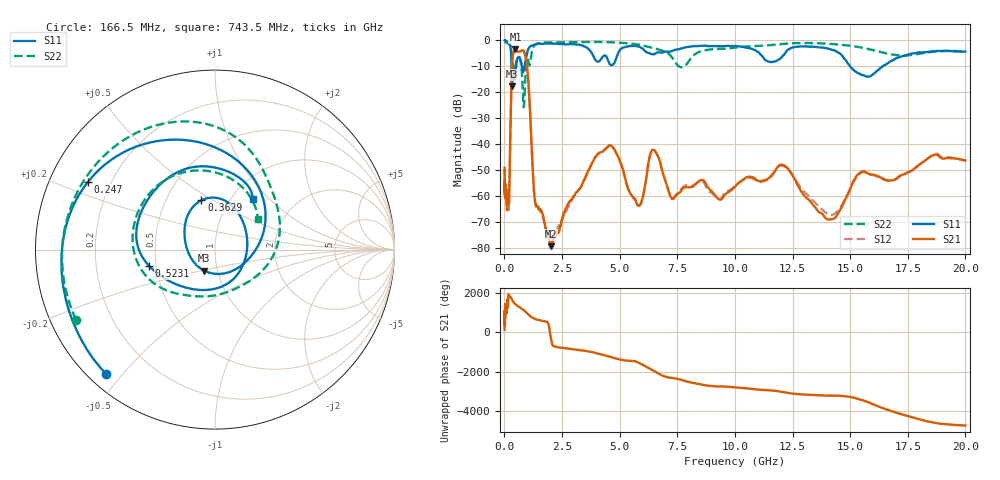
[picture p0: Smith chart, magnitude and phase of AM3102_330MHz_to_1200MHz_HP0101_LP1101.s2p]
! Date/Time: Tue, Sep 11, 2018 5:14 PM
! Network Analyzer: Agilent Technologies E8362B Rev: A.07.50.63
! Sweep from 0.010 to 20.000 GHz, 1601 Points, Sweep Type: LOG
! Power Supply: 4.949 V, 0.001 A
# Hz S DB R 50
!freq MagS11 AngS11 MagS21 AngS21 MagS12 AngS12 MagS22 AngS22
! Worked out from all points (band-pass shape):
!   1601 points, 10 MHz to 20 GHz, reference 50 ohm
!   highest |S21| = -3.47 dB at 478 MHz (marker M1); lowest = -79.2 dB at 2.026 GHz (marker M2)
!   |S21| within 3 dB of the highest: 354.8 MHz to 926.7 MHz (571.8 MHz wide, 89.2 % of centre)
!   lowest |S11| = -17.6 dB at 331.5 MHz (marker M3), VSWR 1.30, Z = 43.2 - j10.4 ohm
!   |S11| at or under -10 dB: 309.5 MHz to 504.8 MHz (195.3 MHz wide, 48 % of centre); 760 MHz to 868.9 MHz (108.9 MHz wide, 13.4 % of centre); 15.01 GHz to 16.41 GHz (1.4 GHz wide, 8.92 % of centre)
!   |S22| runs from -25.7 to -0.3 dB; largest |S21 - S12| = 0.012
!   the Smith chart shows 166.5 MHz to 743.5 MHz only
!   S11 on the Smith chart (normalised r, x): 166.5 MHz: 0.05, -0.45; 247 MHz: 0.12, +0.25; 362.9 MHz: 0.75, +0.45; 523.1 MHz: 0.46, -0.10; 743.5 MHz: 1.24, +0.81
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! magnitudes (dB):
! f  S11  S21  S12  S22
! 10 MHz  0.0  -49.1  -49.4  -0.3
! 35.55 MHz  0.0  -58.7  -58.4  -0.6
! 126.4 MHz  -0.4  -61.5  -63.5  -1.1
! 166.5 MHz  -0.7  -61.7  -64.2  -1.2
! 247 MHz  -1.9  -42.1  -42.2  -1.8
! 331.5 MHz  -17.6  -9.1  -9.1  -5.8
! 362.9 MHz  -10.9  -6.0  -6.1  -8.2
! 447.2 MHz  -14.2  -3.6  -3.6  -11.9
! 478 MHz  -12.4  -3.5  -3.5  -10.7
! 523.1 MHz  -8.5  -3.7  -3.9  -8.2
! 743.5 MHz  -9.0  -3.9  -4.0  -10.7
! 837.2 MHz  -11.6  -4.1  -4.2  -25.7
! 988.7 MHz  -4.6  -10.5  -10.5  -7.4
! 1.302 GHz  -1.6  -59.8  -60.7  -1.9
! 1.59 GHz  -1.3  -65.7  -66.1  -0.9
! 2.026 GHz  -1.2  -79.2  -78.2  -0.8
! 4.5 GHz  -7.7  -40.9  -40.8  -0.6
! 5.652 GHz  -2.1  -61.0  -61.4  -1.4
! 6.518 GHz  -5.2  -42.3  -42.6  -3.0
! 12.15 GHz  -5.4  -48.1  -48.6  -1.3
! 14.07 GHz  -3.2  -69.0  -66.9  -1.3
! 20 GHz  -4.3  -46.2  -46.5  -4.2
